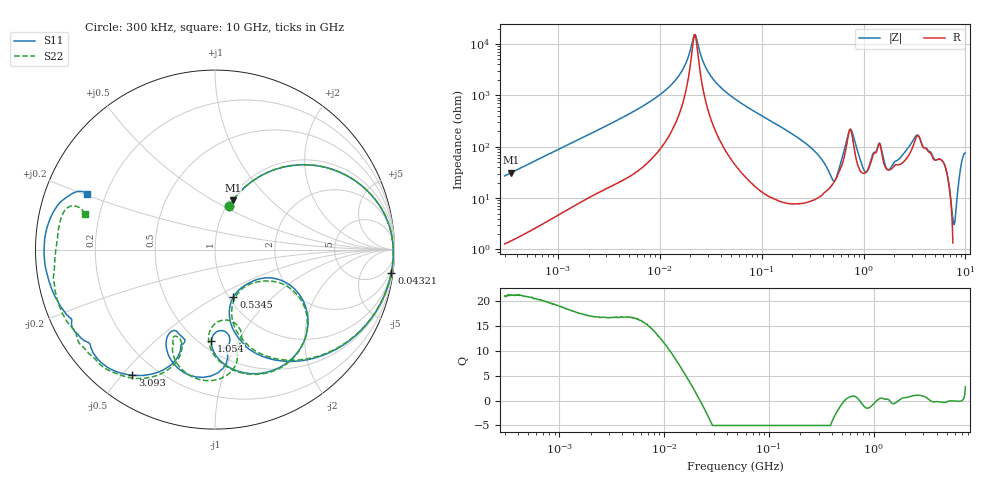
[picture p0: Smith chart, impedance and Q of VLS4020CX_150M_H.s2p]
! S-Parameter Data Generated by TDK Corporation
! Copyright(C) 2024 TDK Corporation.
! All Rights Reserved.
! TDK P/N: VLS4020CX-150M-H (SMD / SMT Inductor (Coil))
! Property: L=15uH at 1MHz
! Size(LxWxT): 4x4x2mm
! Model Type: s2p (Touchstone File Format Version 1.0)
! Frequency: DC=Yes Start=0.3MHz Stop=10000MHz 802points Log-sweep
! Model Generated on May 28, 2024
! Terms and conditions regarding TDK Simulation Models:
! 1)This simulation model is being provided solely for informational
!  purposes. Please refer to the specifications of the products in
!  terms of detailed characteristics of such products.
! 2)In no event shall TDK Corporation of any of its subsidiaries be
!  liable for any loss or damage arising, directly or indirectly,
!  from any information contained in this simulation model, including,
!  but not limited to loss or damages arising from any inaccuracies,
!  omissions or errors in connection with such information.
! 3)Any and all copyrights on this simulation model are owned by
!  TDK Corporation.  Duplication or redistribution of this simulation
!  model without prior written permission from TDK Corporation
!  is prohibited.
! 4)This simulation model is subject to any modification or change
!  without any prior notice.
! 5)Neither TDK Corporation nor any of its subsidiaries shall make any
!  warranty, express or implied, including but not limited to the
!  correctness, implied warranties of merchantability and fitness for
!  a particular purpose with respect to this simulation models.
! 6)The use of this simulation model shall be deemed to have consented
!  to the terms and conditions hereof.
! Port Assignments:
!  1 ---@@@--- 2
! Applicable Conditions:
!  Temperature = 25 degC
!  DC Bias Current = 0 A
!  Small Signal Operation
# Hz S MA R 50
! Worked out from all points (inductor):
!   801 points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, 300 kHz to 10 GHz, reference 50 ohm
!   read as one part in series: L = 14.2 uH near 318.3 kHz
!   highest Q = 21.2 at 345.8 kHz (marker M1), where L = 14.3 uH
!   self-resonance near 21.89 MHz
!   S11 on the Smith chart (normalised r, x): 300 kHz: 1.03, +0.54; 43.21 MHz: 1, -15; 534.5 MHz: 1.05, -0.60; 1.054 GHz: 0.57, -0.78; 3.093 GHz: 0.11, -0.53; 10 GHz: 0.13, +0.21
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300000  0.2562 72.3  0.9544 -15.0  0.9543 -14.9  0.2564 72.3
345843  0.2914 70.2  0.9428 -17.0  0.943 -17.0  0.2914 70.3
1713600  0.8066 32.9  0.5463 -53.7  0.5464 -53.7  0.8065 32.9
9671944  0.9865 5.2  0.1011 -80.1  0.1012 -80.1  0.9865 5.2
1.603896e7  0.9923 1.0  0.03655 -77.9  0.03657 -77.9  0.9924 1.1
2.220835e7  0.9935 -1.5  0.006486 4.5  0.006495 4.6  0.9935 -1.4
2.856806e7  0.9933 -3.5  0.02965 74.6  0.02965 74.5  0.9934 -3.4
4.320848e7  0.9908 -7.4  0.08077 78.4  0.0808 78.4  0.9908 -7.3
5.477226e7  0.9872 -10.2  0.1157 76.9  0.1158 76.9  0.9872 -10.0
1.405283e8  0.932 -28.5  0.3327 59.8  0.3328 59.8  0.9318 -28.1
3.126428e8  0.7144 -60.0  0.6417 25.9  0.6418 25.9  0.7153 -59.0
5.344909e8  0.2837 -68.9  0.7769 -20.5  0.777 -20.5  0.2864 -66.3
6.325141e8  0.3704 -25.7  0.6177 -45.2  0.6177 -45.2  0.4034 -27.3
7.152593e8  0.6674 -39.1  0.3206 -48.0  0.3206 -48.0  0.6809 -41.1
8.414386e8  0.7278 -71.8  0.4302 -8.1  0.4302 -8.1  0.7266 -73.2
1.054047e9  0.5084 -92.2  0.6349 -35.4  0.6351 -35.4  0.4785 -94.2
1.339606e9  0.5511 -84.3  0.4349 -63.4  0.4352 -63.4  0.5754 -77.7
1.767019e9  0.5712 -118.3  0.506 -62.1  0.5063 -62.1  0.6153 -112.6
2.446702e9  0.6119 -108.9  0.3911 -112.2  0.3909 -112.3  0.5805 -108.5
3.093017e9  0.8385 -123.4  0.1524 -141.6  0.1522 -141.6  0.8356 -120.7
7.222042e9  0.9509 -174.6  0.06651 -125.1  0.06652 -125.1  0.9143 -170.2
1e10  0.7809 156.5  0.04724 -125.1  0.04731 -125.2  0.7496 164.5
